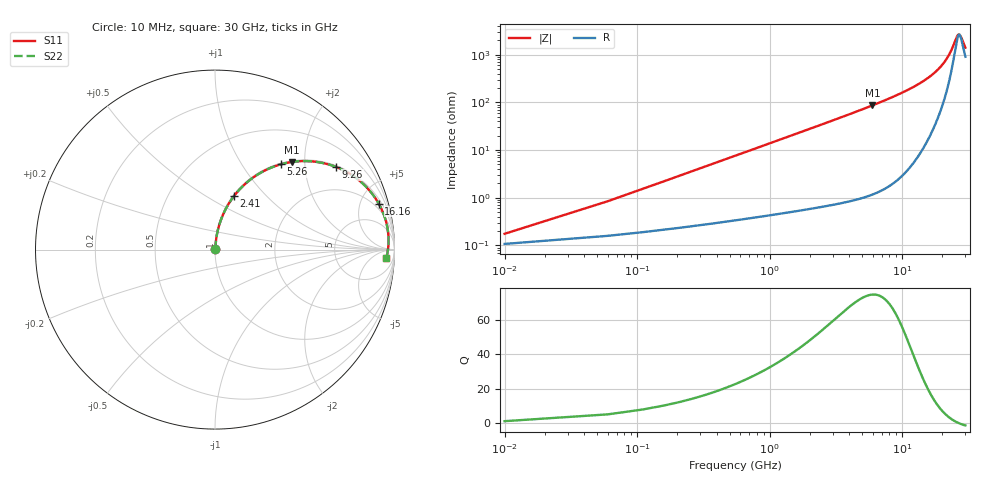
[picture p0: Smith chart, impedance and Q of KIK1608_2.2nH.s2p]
!version-2
!date-01.2022
!Series
# MHz S RI R 50
!Freq ReS11 ImS11 ReS21 ImS21 ReS12 ImS12 ReS22 ImS22
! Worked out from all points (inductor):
!   601 points, 10 MHz to 30 GHz, reference 50 ohm
!   read as one part in series: L = 2.2 nH near 160 MHz
!   highest Q = 74.5 at 5.96 GHz (marker M1), where L = 2.31 nH
!   self-resonance near 27.05 GHz
!   S11 on the Smith chart (normalised r, x): 10 MHz: 1.00, +0.00; 2.41 GHz: 1.01, +0.67; 5.26 GHz: 1.02, +1.51; 9.26 GHz: 1.05, +2.91; 16.16 GHz: 1.39, +6.97; 30 GHz: 19, -22
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10  0.00107 0.00138  0.9989 -0.00138  0.9989 -0.00138  0.00107 0.00138
210  0.00317 0.0289  0.9968 -0.0289  0.9968 -0.0289  0.00317 0.0289
260  0.0038 0.0357  0.9962 -0.0357  0.9962 -0.0357  0.0038 0.0357
410  0.00615 0.0562  0.9938 -0.0562  0.9938 -0.0562  0.00615 0.0562
560  0.00926 0.0765  0.9907 -0.0765  0.9907 -0.0765  0.00926 0.0765
860  0.0178 0.1164  0.9822 -0.1164  0.9822 -0.1164  0.0178 0.1164
1260  0.0339 0.1679  0.9661 -0.1679  0.9661 -0.1679  0.0339 0.1679
2410  0.1059 0.2984  0.8941 -0.2984  0.8941 -0.2984  0.1059 0.2984
3560  0.2043 0.3955  0.7957 -0.3955  0.7957 -0.3955  0.2043 0.3955
5010  0.342 0.4675  0.658 -0.4675  0.658 -0.4675  0.342 0.4675
5260  0.3656 0.4748  0.6344 -0.4748  0.6344 -0.4748  0.3656 0.4748
5960  0.4299 0.4884  0.5701 -0.4884  0.5701 -0.4884  0.4299 0.4884
9260  0.6759 0.4599  0.3241 -0.4599  0.3241 -0.4599  0.6759 0.4599
10010  0.7174 0.4414  0.2826 -0.4414  0.2826 -0.4414  0.7174 0.4414
15010  0.8904 0.2911  0.1096 -0.2911  0.1096 -0.2911  0.8904 0.2911
16160  0.9119 0.2567  0.0881 -0.2567  0.0881 -0.2567  0.9119 0.2567
20010  0.9543 0.1513  0.0457 -0.1513  0.0457 -0.1513  0.9543 0.1513
22660  0.9652 0.0884  0.0348 -0.0884  0.0348 -0.0884  0.9652 0.0884
25010  0.9668 0.0387  0.0332 -0.0387  0.0332 -0.0387  0.9668 0.0387
26160  0.9655 0.0165  0.0345 -0.0165  0.0345 -0.0165  0.9655 0.0165
27010  0.9637 0.000786  0.0363 -0.000786  0.0363 -0.000786  0.9637 0.000786
30000  0.9537 -0.0494  0.0463 0.0494  0.0463 0.0494  0.9537 -0.0494
